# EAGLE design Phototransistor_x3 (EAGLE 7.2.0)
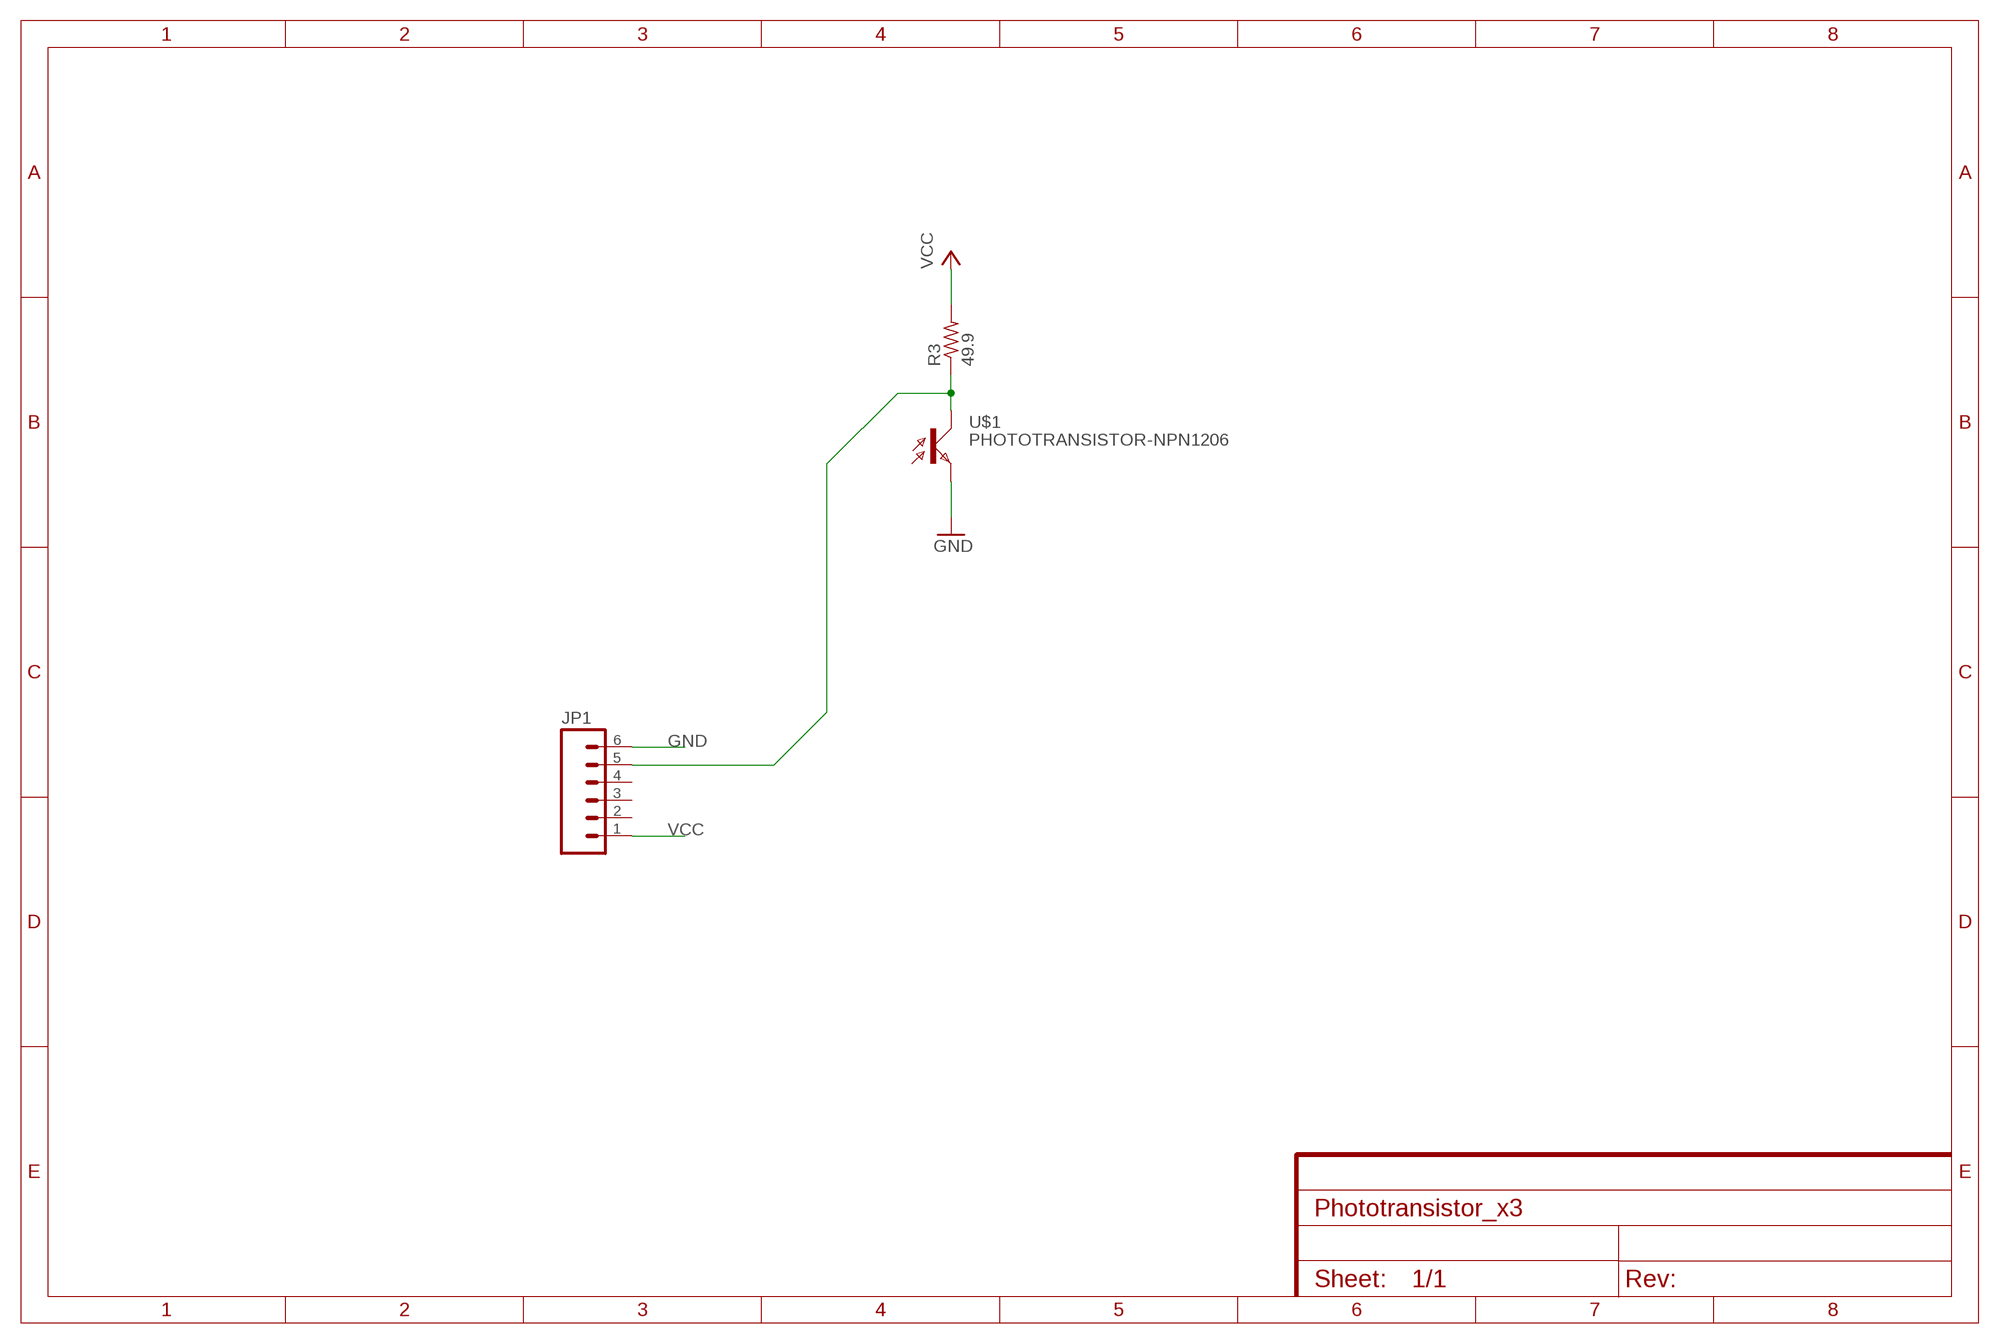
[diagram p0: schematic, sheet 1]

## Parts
JP1  M06SMD  [1X06-SMD]
R3  49.9  RESISTOR1206  [1206]
U$1  PHOTOTRANSISTOR-NPN1206  [OP1206]

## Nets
GND: JP1.6 U$1.EMITTER(E)
N$3: JP1.5 R3.1 U$1.COLLECTOR(C)
VCC: JP1.1 R3.2
Unconnected: JP1.2 JP1.3 JP1.4

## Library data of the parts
JP1 = SparkFun:M06: Header 6 Standard 6-pin 0.1" header. Use with straight break away headers (SKU : PRT-00116), right angle break away headers (PRT-00553), swiss pins (PRT-00743), machine pins (PRT-00117), and female headers (PRT-00115). Molex polarized connector foot print use with SKU : PRT-08094 with associated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
R3 = 01_ng:RESISTOR
U$1 = 01_fab:PHOTOTRANSISTOR-NPN

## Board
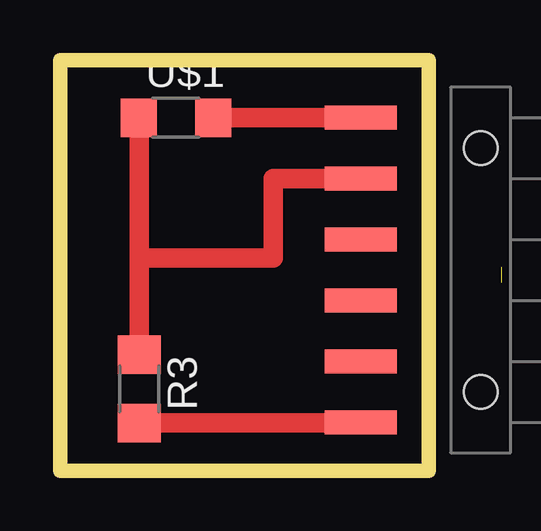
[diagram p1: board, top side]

Size 15.37 x 17.14 mm. Coordinates in mm from the lower left corner, seen from the top.
Outline: 0,0 15.37,0 15.37,17.14 0,17.14 0,0
Copper layers 1: Top 0.035mm
Design rules "ERP-1sided-10mil-16mill *": minimum track width 16mil, minimum drill 24mil, track to track 16mil, track to pad 16mil, pad to pad 16mil, via to via 16mil, smd to smd 0mil, copper to edge 16mil, drill to drill 36mil, minimum pad ring 10mil, minimum via ring 8mil, stop-mask expansion 4mil, vias tented up to drill 0mil, thermal gap 10mil

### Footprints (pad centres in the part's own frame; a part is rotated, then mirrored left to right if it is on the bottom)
1X06-SMD = smd 1 x 3: 1 -6.35,5; 2 -3.81,5; 3 -1.27,5; 4 1.27,5; 5 3.81,5; 6 6.35,5 | hole 1.4: -5.08,0; 5.08,0
1206 = smd 1.6 x 1.803: 1 -1.422,0; 2 1.422,0
OP1206 = smd 1.5 x 1.6: COLLECTOR -1.55,0; EMITTER 1.55,0

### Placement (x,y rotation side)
JP1  17.53,8.38 90 top
R3  3.3,3.43 270 top
U$1  4.83,14.73 0 top

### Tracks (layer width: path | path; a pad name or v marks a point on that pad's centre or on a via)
GND
  Top 0.813: U$1.EMITTER JP1.6
N$3
  Top 0.813: U$1.COLLECTOR 3.3,14.73 3.3,8.89 | R3.1 3.3,8.76 3.3,8.89 | JP1.5 8.89,12.19 8.89,8.89 3.3,8.89
N$15  (1 unrouted)
VCC
  Top 0.813: R3.2 12.53,2.01 JP1.1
